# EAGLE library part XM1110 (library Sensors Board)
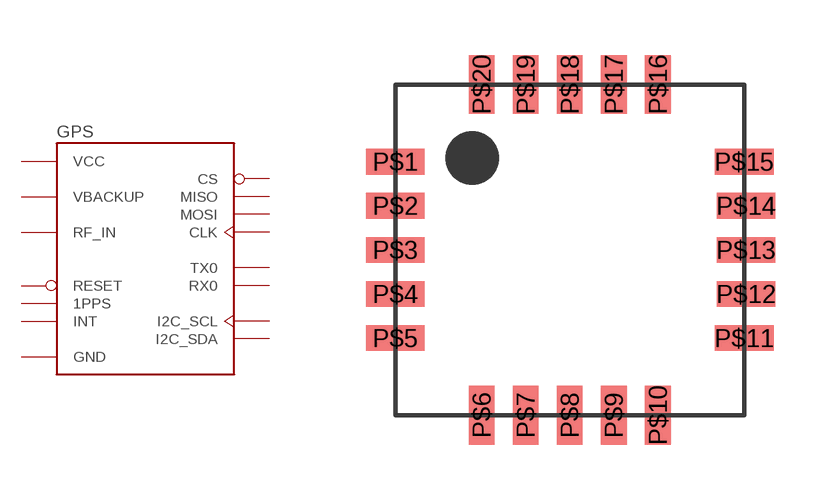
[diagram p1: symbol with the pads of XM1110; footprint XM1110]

Designator prefix GPS

## XM1110  [XM1110]
P$1  GND  sup
P$2  RF_IN  in
P$3  GND  sup
P$4  GND  sup
P$5  GND  sup
P$6  GND  sup
P$7  VCC  sup
P$8  VBACKUP  sup
P$9  GND  sup
P$10  I2C_SDA
P$11  I2C_SCL  in
P$12  MISO  out
P$13  INT  out
P$14  MOSI  in
P$15  CLK  in
P$16  TX0  out
P$17  RX0  in
P$18  1PPS  out
P$19  RESET  in
P$20  CS  in

## Footprint XM1110 (pad centres in mm)
smd 1.6 x 0.7: P$1 -4.75,2.4; P$2 -4.75,1.2; P$3 -4.75,0; P$4 -4.75,-1.2; P$5 -4.75,-2.4; P$11 4.75,-2.4; P$12 4.8,-1.2; P$13 4.8,0; P$14 4.8,1.2; P$15 4.75,2.4
smd 0.7 x 1.6: P$6 -2.4,-4.5; P$7 -1.2,-4.5; P$8 0,-4.5; P$9 1.2,-4.5; P$10 2.4,-4.5; P$16 2.4,4.5; P$17 1.2,4.5; P$18 0,4.5; P$19 -1.2,4.5; P$20 -2.4,4.5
